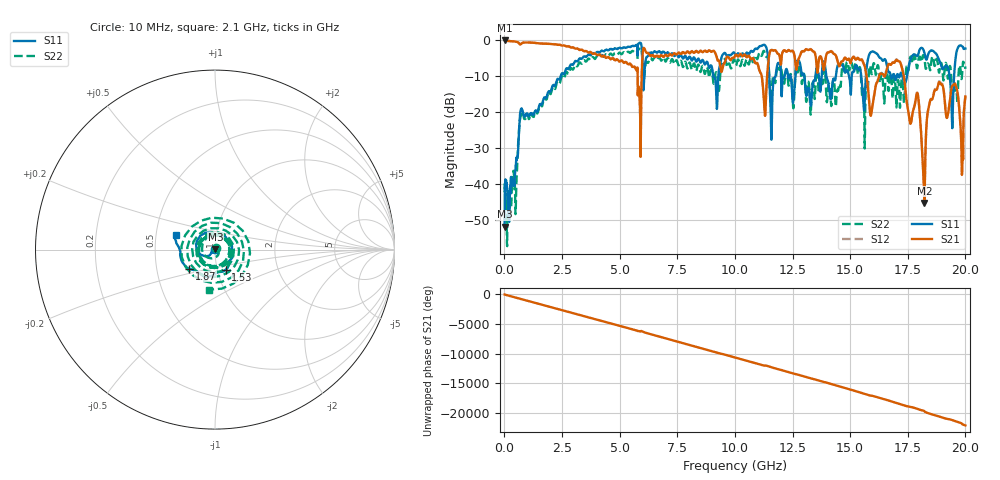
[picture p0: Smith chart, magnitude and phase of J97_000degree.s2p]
!Keysight Technologies,N5222A,MY51421036,A.10.65.16
!Date: Friday, March 31, 2023 14:29:46
!Correction: S11(Full 2 Port(1,2))
!S21(Full 2 Port(1,2))
!S12(Full 2 Port(1,2))
!S22(Full 2 Port(1,2))
!S2P File: Measurements: S11, S21, S12, S22:
# Hz S  dB  R 50
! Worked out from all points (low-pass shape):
!   2000 points, 10 MHz to 20 GHz, reference 50 ohm
!   highest |S21| = -0.02 dB at 10 MHz (marker M1); lowest = -45.3 dB at 18.22 GHz (marker M2)
!   |S21| within 3 dB of the highest: start of sweep to 3.454 GHz; 13.01 GHz to 13.38 GHz (377.8 MHz wide, 2.86 % of centre)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
!   lowest |S11| = -51.9 dB at 10 MHz (marker M3), VSWR 1.01, Z = 50.2 + j0.169 ohm
!   |S11| at or under -10 dB: start of sweep to 2.444 GHz; 13.01 GHz to 13.5 GHz (483.8 MHz wide, 3.65 % of centre); 13.97 GHz to 14.38 GHz (412.3 MHz wide, 2.91 % of centre)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
!   |S22| runs from -57.4 to -2.0 dB; largest |S21 - S12| = 0.013
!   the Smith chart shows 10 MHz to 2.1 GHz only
!   S11 on the Smith chart (normalised r, x): 10 MHz: 1.00, +0.00; 1.53 GHz: 1.10, -0.25; 1.87 GHz: 0.73, -0.16; 2.1 GHz: 0.63, +0.11
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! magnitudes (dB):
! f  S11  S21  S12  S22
! 10 MHz  -51.9  0.0  -0.1  -39.9
! 450 MHz  -38.3  -0.3  -0.3  -39.4
! 740 MHz  -19.1  -0.9  -0.9  -20.0
! 1.53 GHz  -18.0  -0.9  -0.8  -17.9
! 1.87 GHz  -15.0  -1.0  -0.9  -15.5
! 2.1 GHz  -12.6  -1.1  -1.0  -12.9
! 3.35 GHz  -5.1  -2.6  -2.5  -6.5
! 5.86 GHz  -0.7  -15.0  -15.0  -2.4
! 6.68 GHz  -3.1  -4.6  -4.5  -4.8
! 10.01 GHz  -3.9  -4.2  -4.3  -6.3
! 11.29 GHz  -1.2  -19.8  -19.8  -3.3
! 11.59 GHz  -27.7  -2.7  -2.7  -14.3
! 13.34 GHz  -14.8  -2.8  -2.7  -13.5
! 15.47 GHz  -9.3  -5.4  -5.3  -10.1
! 15.92 GHz  -3.2  -20.4  -20.4  -9.1
! 16.67 GHz  -8.9  -6.6  -6.5  -14.1
! 17.92 GHz  -4.3  -14.8  -14.6  -7.5
! 18.22 GHz  -3.4  -45.3  -45.1  -4.9
! 18.81 GHz  -4.7  -12.6  -12.4  -6.8
! 19.41 GHz  -20.8  -12.9  -12.7  -13.6
! 19.83 GHz  -1.5  -30.7  -30.7  -10.8
! 20 GHz  -2.3  -15.7  -15.4  -7.9
